[IBIS Ver]   4.1
[File Name]   tms570ls31x_21x_revb_zwt.ibs
[File Rev]   1.0
[Date]   Tue Aug 20 12:42:00 2013
[Source]   Texas Instruments, Inc.
[Notes]   Revision History:
   1.0: initial release, 08/20/2013
   THIS IS RELEASE 1.0,THE CONTENTS ARE SUBJECT TO
   CHANGE WITHOUT PRIOR NOTICE,IF NECESSARY.
[Disclaimer] Please be aware that in the absence of a written agreement
   Texas Instruments(TI) assumes no liability for:
   (1) The accuracy of the IBIS models provided to your company
   (2) The proper functioning of these Models in your design
   or for any resulting applications;or
   (3) Infringement of patents,copyrights or intellectual
   property rights resulting from your use of these models.
   TI provides IBIS Models as a service to our customers and
   therefore reserves the right to limit distribution of the
   Models.
[Copyright]   Property of Texas Instruments Incorporated.
   Unauthorised reproduction and/or distribution is strictly.
   prohibited.
   This product is protected under copyright law and trade
   secret law as an unpublished work.
   Created 2013,(C) Copyright 2013-2014,
   Texas Instruments Incorporated., All Rights Reserved.
   These commodities are under the U.S. Government
   distribution license control.As such,they are not to be
   re-exported without the prior approval of the
   U.S. Department of Commerce.
[Component]   TMS570LS31x/21xZWT
[Manufacturer]   Texas Instruments
[Package]
| variable   typ   min   max
R_pkg   196.67m   3.54953m   570.977m
L_pkg   4.5808nH   0.0479255nH   19.1106nH
C_pkg   1.53489pF   0.703339pF   29.6807pF
[Pin]   signal_name   model_name   R_pin   L_pin   C_pin
|N19	AD1EVT   BQ0210FT	184.966m	4.32413nH	0.998379pF
|V17	AD1IN[01]   IQ0078FT5	151.205m	3.61421nH	1.06433pF
|V18	AD1IN[02]   IQ0078FT5	162.921m	4.0194nH	1.09587pF
|T17	AD1IN[03]   IQ0078FT5	132.107m	2.87623nH	1.02282pF
|U18	AD1IN[04]   IQ0078FT5	150.378m	3.74239nH	0.871765pF
|R17	AD1IN[05]   IQ0078FT5	121.29m   2.64503nH	0.889504pF
|T19	AD1IN[06]   IQ0078FT5	160.561m	4.24427nH	0.832099pF
|V14	AD1IN[07]   IQ0078FT5	124.5m   2.801nH   0.801931pF
|P18	AD1IN[08]_AD2IN[08]	IQ0444FT5	168.416m	3.58257nH	0.854547pF
|W17	AD1IN[09]_AD2IN[09]	IQ0444FT5	176.52m   4.34386nH	0.998673pF
|W14	AD1IN[0]   IQ0078FT5	144.705m	3.56911nH	0.794686pF
|U17	AD1IN[10]_AD2IN[10]	IQ0444FT5	144.94m   3.19721nH	0.980765pF
|U19	AD1IN[11]_AD2IN[11]	IQ0444FT5	171.775m	4.43186nH	0.907619pF
|T16	AD1IN[12]_AD2IN[12]	IQ0444FT5	125.156m	2.59352nH	0.876512pF
|T18	AD1IN[13]_AD2IN[13]	IQ0444FT5	144.177m	3.64898nH	0.839357pF
|R18	AD1IN[14]_AD2IN[14]	IQ0444FT5	165.024m	3.55051nH	0.817191pF
|P19	AD1IN[15]_AD2IN[15]	IQ0444FT5	182.297m	4.13942nH	0.76377pF
|V13	AD1IN[16]_AD2IN[0]	IQ0444FT5	120.853m	2.65468nH	0.725617pF
|U13	AD1IN[17]_AD2IN[01]	IQ0444FT5	100.582m	1.89517nH	0.782711pF
|U14	AD1IN[18]_AD2IN[02]	IQ0444FT5	126.715m	2.5688nH	0.798277pF
|U16	AD1IN[19]_AD2IN[03]	IQ0444FT5	178.504m	4.50312nH	0.988444pF
|U15	AD1IN[20]_AD2IN[04]	IQ0444FT5	119.937m	2.69452nH	0.835124pF
|T15	AD1IN[21]_AD2IN[05]	IQ0444FT5	112.602m	2.37779nH	0.929566pF
|R19	AD1IN[22]_AD2IN[06]	IQ0444FT5	182.419m	4.23756nH	0.798392pF
|R16	AD1IN[23]_AD2IN[07]	IQ0444FT5	142.476m	2.71607nH	0.906429pF
|V15	ADREFHI   BAFTHRU50FT	119.48m		2.9557nH	0.922653pF
|V16	ADREFLO   BAFTHRU50FT	131.598m	3.42945nH	1.00012pF
B10	CAN1RX   BQ0210FT	372.361m	9.36494nH	2.26135pF
A10	CAN1TX			BQ0210FT	363.638m	9.59412nH	2.23947pF
H1	CAN2RX			BQ0210FT	469.673m	12.1979nH	2.87424pF
H2	CAN2TX			BQ0210FT	470.032m	15.4394nH	2.57149pF
M19	CAN3RX			BQ0210FT	401.594m	9.66373nH	2.44197pF
M18	CAN3TX			BQ0210FT	391.963m	9.46214nH	2.55062pF
F17	DMM_CLK			BQ0210FT	153.912m	2.83152nH	1.05028pF
L19	DMM_DATA[0]		BQ0210FT	228.208m	5.86168nH	1.10015pF
L18	DMM_DATA[1]		BQ0210FT	152.021m	3.20684nH	0.961632pF
F16	DMM_NENA		BQ0210FT	109.558m	1.97175nH	1.01071pF
J16	DMM_SYNC		BQ0210FT	131.945m	2.28134nH	1.06088pF
A12	ECLK			BQ0215FT	148.114m	3.69152nH	0.965063pF
D4	EMIF_ADDR[0]		BQ0212FT	205.844m	4.75509nH	1.59007pF
C8	EMIF_ADDR[10]		BQ0212FT	238.21m		5.83758nH	1.71133pF
C9	EMIF_ADDR[11]		BQ0212FT	128.313m	2.08531nH	0.871154pF
C10	EMIF_ADDR[12]		BQ0212FT	123.215m	1.9766nH	0.84691pF
C11	EMIF_ADDR[13]		BQ0212FT	159.315m	3.04056nH	0.957165pF
C12	EMIF_ADDR[14]		BQ0212FT	118.286m	2.54469nH	0.890332pF
C13	EMIF_ADDR[15]		BQ0212FT	126.478m	2.95876nH	0.982603pF
D14	EMIF_ADDR[16]		BQ0212FT	145.307m	2.51953nH	0.973601pF
C14	EMIF_ADDR[17]		BQ0212FT	120.672m	2.47733nH	0.940052pF
D15	EMIF_ADDR[18]		BQ0212FT	111.953m	2.31215nH	0.945399pF
C15	EMIF_ADDR[19]		BQ0212FT	118.554m	2.38397nH	0.981384pF
D5	EMIF_ADDR[1]		BQ0212FT	197.193m	4.27023nH	1.42867pF
C16	EMIF_ADDR[20]		BQ0212FT	150.887m	2.83734nH	1.20313pF
C17	EMIF_ADDR[21]		BQ0212FT	176.774m	3.69908nH	1.27863pF
C4	EMIF_ADDR[6]		BQ0215FT	278.52m   8.56148nH	1.69347pF
C5	EMIF_ADDR[7]		BQ0215FT	304.187m	5.90295nH	2.18684pF
C6	EMIF_ADDR[8]		BQ0215FT	307.858m	6.87831nH	2.13437pF
C7	EMIF_ADDR[9]		BQ0212FT	194.675m	3.98027nH	1.28957pF
D16	EMIF_BA[1]		BQ0215FT	195.47m   4.24161nH	1.29408pF
L3	EMIF_CKE		BQ0212FT	141.86m   2.6218nH	0.864293pF
K3	EMIF_CLK		BQ0212FT	156.267m	3.34722nH	1.22338pF
R4	EMIF_NCAS		BQ0212FT	114.553m	2.02583nH	1.04824pF
N17	EMIF_NCS[0]		BQ0215FT	138.476m	2.73863nH	0.941691pF
L17	EMIF_NCS[2]		BQ0212FT	130.559m	2.55792nH	0.959974pF
K17	EMIF_NCS[3]		BQ0215FT	149.052m	2.77825nH	0.971145pF
M17	EMIF_NCS[4]		BQ0212FT	191.312m	4.44479nH	1.32158pF
R3	EMIF_NRAS		BQ0212FT	148.328m	2.95135nH	1.02744pF
P3	EMIF_NWAIT		BQ0212FT	183.791m	3.30593nH	0.996769pF
D17	EMIF_NWE		BQ0212FT	253.876m	6.55734nH	1.26073pF
R13	ETMDATA[01]		BQ0212FT	124.479m	2.37232nH	0.870061pF
J15	ETMDATA[02]		BQ0212FT	103.911m	1.27754nH	0.953532pF
H15	ETMDATA[03]		BQ0212FT	87.7259m	1.35214nH	1.02626pF
G15	ETMDATA[04]		BQ0212FT	141.552m	2.19702nH	1.13315pF
F15	ETMDATA[05]		BQ0212FT	108.038m	2.13506nH	1.1894pF
E15	ETMDATA[06]		BQ0212FT	150.765m	2.54749nH	1.22031pF
E14	ETMDATA[07]		BQ0212FT	114.504m	1.75736nH	1.21873pF
E9	ETMDATA[08]		BQ0212FT	109.16m   1.64189nH	1.10519pF
E8	ETMDATA[09]		BQ0212FT	144.452m	2.94238nH	1.14497pF
R12	ETMDATA[0]		BQ0212FT	83.6868m	0.985017nH	0.869529pF
E7	ETMDATA[10]		BQ0212FT	214.54m   4.14551nH	1.13678pF
E6	ETMDATA[11]		BQ0212FT	182.856m	3.65155nH	1.40417pF
E13	ETMDATA[12]		BQ0212FT	77.0047m	0.812185nH	0.977195pF
E12	ETMDATA[13]		BQ0212FT	138.149m	1.98855nH	0.973006pF
E11	ETMDATA[14]		BQ0212FT	119.216m	1.28477nH	0.922331pF
E10	ETMDATA[15]		BQ0212FT	118.762m	1.28027nH	0.875094pF
K15	ETMDATA[16]		BQ0212FT	105.18m   1.27303nH	0.910587pF
L15	ETMDATA[17]		BQ0212FT	108.292m	1.30922nH	0.956891pF
M15	ETMDATA[18]		BQ0212FT	146.648m	3.23796nH	1.11212pF
N15	ETMDATA[19]		BQ0212FT	151.481m	2.39079nH	1.04051pF
E5	ETMDATA[20]		BQ0212FT	240.049m	4.95227nH	1.34761pF
F5	ETMDATA[21]		BQ0212FT	200.894m	3.43241nH	1.2936pF
G5	ETMDATA[22]		BQ0212FT	113.089m	1.56898nH	1.27784pF
K5	ETMDATA[23]		BQ0212FT	159.632m	2.73815nH	1.23965pF
L5	ETMDATA[24]		BQ0212FT	107.976m	1.33411nH	0.987891pF
M5	ETMDATA[25]		BQ0212FT	158.798m	1.84169nH	0.949294pF
N5	ETMDATA[26]		BQ0212FT	104.885m	1.27901nH	0.956427pF
P5	ETMDATA[27]		BQ0212FT	111.148m	1.31516nH	0.975979pF
R5	ETMDATA[28]		BQ0212FT	99.3475m	1.3689nH	1.06642pF
R6	ETMDATA[29]		BQ0212FT	97.4645m	1.43736nH	1.09879pF
R7	ETMDATA[30]		BQ0212FT	124.403m	1.9796nH	0.99492pF
R8	ETMDATA[31]		BQ0212FT	104.139m	1.40991nH	0.846212pF
R9	ETMTRACECLKIN		BQ0212FT	121.779m	1.22371nH	0.853714pF
R10	ETMTRACECLKOUT		BQ0212FT	142.063m	1.98785nH	0.918845pF
R11	ETMTRACECTL		BQ0212FT	190.384m	2.91831nH	0.965226pF
|J5	FLTP1			BAFTHRU15VFT   149.492m	2.20118nH	1.45838pF
|H5	FLTP2			BAFTHRU8VFT   165.991m	2.9168nH	1.52069pF
A15	FRAYRX1			IQ0442FT_40P60P	239.448m	7.10463nH	1.25424pF
A8	FRAYRX2			IQ0442FT_40P60P	258.134m	7.31683nH	1.55084pF
B15	FRAYTX1			OQ0112FT	304.358m	8.80599nH	1.6535pF
B8	FRAYTX2			OQ0112FT	226.744m	5.13131nH	1.43502pF
B16	FRAYTXEN1		OQ0112FT	349.226m	11.4289nH	1.99559pF
B9	FRAYTXEN2		OQ0112FT	258.966m	6.63073nH	1.55419pF
A5	GIOA[0]			BQ0210FT	190.079m	4.2665nH	1.13619pF
C2	GIOA[1]			BQ0210FT	185.052m	4.37032nH	1.10133pF
C1	GIOA[2]			BQ0215FT	218.526m	6.21769nH	1.17667pF
E1	GIOA[3]			BQ0210FT	210.54m   5.74448nH	1.10806pF
A6	GIOA[4]			BQ0210FT	385.739m	11.963nH	2.08522pF
B5	GIOA[5]			BQ0210FT	280.374m	5.73605nH	2.17708pF
H3	GIOA[6]			BQ0210FT	161.443m	4.06305nH	1.16964pF
M1	GIOA[7]			BQ0210FT	216.429m	4.60646nH	0.861283pF
M2	GIOB[0]			BQ0215FT	344.684m	8.17302nH	2.2998pF
K2	GIOB[1]			BQ0215FT	513.961m	16.8626nH	2.48021pF
F2	GIOB[2]			BQ0210FT	256.042m	6.4832nH	1.48887pF
W10	GIOB[3]			BQ0210FT	564.754m	12.7444nH	3.11943pF
G1	GIOB[4]			BQ0210FT	207.863m	4.2053nH	1.17746pF
G2	GIOB[5]			BQ0210FT	176.17m   4.21454nH	1.07738pF
J2	GIOB[6]			BQ0210FT	249.666m	4.98691nH	1.1261pF
F1	GIOB[7]			BQ0210FT	431.321m	11.1455nH	2.1899pF
|L2	KELVIN_GND		GND   144.49m   3.36085nH	0.855052pF
A7	LINRX			BQ0210FT	164.093m	3.51713nH	0.789652pF
B7	LINTX			BQ0210FT	149.514m	3.76138nH	0.974205pF
F18	MIBSPI1CLK		BQ0211FT	209.432m	5.11407nH	1.36171pF
R2	MIBSPI1NCS[0]		BQ0215FT	438.232m	9.65193nH	2.73624pF
F3	MIBSPI1NCS[1]		BQ0215FT	249.337m	5.36744nH	1.38728pF
G3	MIBSPI1NCS[2]		BQ0215FT	570.977m	19.1106nH	3.13273pF
J3	MIBSPI1NCS[3]		BQ0210FT	533.925m	18.0739nH	2.91425pF
G19	MIBSPI1NENA		BQ0210FT	222.255m	5.67898nH	1.17997pF
F19	MIBSPI1SIMO		BQ0211FT	255.952m	7.3408nH	1.63182pF
G18	MIBSPI1SOMI		BQ0211FT	248.638m	6.78288nH	1.35142pF
V9	MIBSPI3CLK		BQ0211FT	143.966m	2.67746nH	0.710513pF
V10	MIBSPI3NCS[0]		BQ0210FT	159.677m	2.96343nH	0.703339pF
V5	MIBSPI3NCS[1]		BQ0215FT	129.845m	2.82102nH	0.865993pF
B2	MIBSPI3NCS[2]		BQ0210FT	197.146m	4.5376nH	1.01987pF
C3	MIBSPI3NCS[3]		BQ0210FT	173.194m	3.67063nH	1.03815pF
W9	MIBSPI3NENA		BQ0210FT	174.924m	3.75475nH	0.75194pF
W8	MIBSPI3SIMO		BQ0211FT	174.737m	3.8999nH	0.788207pF
V8	MIBSPI3SOMI		BQ0211FT	157.163m	3.04464nH	0.770715pF
H19	MIBSPI5CLK		BQ0212FT	172.551m	4.02962nH	1.0456pF
E19	MIBSPI5NCS[0]		BQ0210FT	434.627m	9.75226nH	2.8982pF
B6	MIBSPI5NCS[1]		BQ0210FT	125.385m	2.81804nH	0.998305pF
W6	MIBSPI5NCS[2]		BQ0210FT	137.701m	3.4368nH	0.777293pF
T12	MIBSPI5NCS[3]		BQ0210FT	88.9463m	1.39nH   0.752235pF
H18	MIBSPI5NENA		BQ0210FT	172.956m	3.92446nH	1.06336pF
J19	MIBSPI5SIMO[0]		BQ0212FT	230.569m	5.55483nH	1.25878pF
E16	MIBSPI5SIMO[1]		BQ0212FT	113.502m	2.01142nH	1.12975pF
H17	MIBSPI5SIMO[2]		BQ0212FT	147.332m	2.72568nH	1.04308pF
G17	MIBSPI5SIMO[3]		BQ0212FT	136.981m	2.49108nH	1.02895pF
J18	MIBSPI5SOMI[0]		BQ0212FT	150.574m	3.17152nH	1.01665pF
E17	MIBSPI5SOMI[1]		BQ0212FT	228.929m	5.42812nH	1.37918pF
H16	MIBSPI5SOMI[2]		BQ0212FT	140.961m	3.01931nH	1.21316pF
G16	MIBSPI5SOMI[3]		BQ0212FT	112.489m	1.67887nH	1.04781pF
B14	NERROR			BQ0212FT	138.758m	3.33213nH	1.04178pF
V2	NHET1[01]		BQ0215FT	338.409m	9.38218nH	1.48365pF
W5	NHET1[02]		BQ0215FT	248.268m	6.84186nH	1.56548pF
U1	NHET1[03]		BQ0215FT	293.29m   7.89763nH	1.33136pF
B12	NHET1[04]		BQ0210FT	384.915m	8.28491nH	2.24703pF
V6	NHET1[05]		BQ0215FT	222.182m	5.35492nH	1.44554pF
W3	NHET1[06]		BQ0210FT	169.477m	4.54954nH	0.866005pF
T1	NHET1[07]		BQ0215FT	177.683m	4.12802nH	0.940453pF
E18	NHET1[08]		BQ0215FT	169.207m	3.50595nH	1.02982pF
V7	NHET1[09]		BQ0215FT	164.378m	3.85974nH	1.41149pF
K18	NHET1[0]		BQ0215FT	502.921m	10.4825nH	2.67359pF
D19	NHET1[10]		BQ0215FT	284.952m	7.64309nH	1.46318pF
E3	NHET1[11]		BQ0210FT	142.81m   2.72692nH	1.13821pF
B4	NHET1[12]		BQ0210FT	363.144m	10.8745nH	1.72677pF
N2	NHET1[13]		BQ0210FT	272.616m	7.56634nH	1.52295pF
A11	NHET1[14]		BQ0215FT	171.543m	3.6018nH	0.779645pF
N1	NHET1[15]		BQ0210FT	279.581m	8.1671nH	1.60856pF
A4	NHET1[16]		BQ0210FT	175.761m	4.52014nH	1.03411pF
A13	NHET1[17]		BQ0210FT	241.835m	6.51525nH	1.41446pF
J1	NHET1[18]		BQ0210FT	265.215m	6.2119nH	2.32332pF
B13	NHET1[19]		BQ0210FT	156.895m	3.0638nH	0.861316pF
P2	NHET1[20]		BQ0210FT	312.077m	7.55077nH	2.22707pF
H4	NHET1[21]		BQ0210FT	111.925m	1.75875nH	1.25067pF
B3	NHET1[22]		BQ0215FT	350.67m   11.5381nH	1.82498pF
J4	NHET1[23]		BQ0210FT	123.48m   1.96598nH	1.02514pF
P1	NHET1[24]		BQ0210FT	396.061m	10.0857nH	2.38747pF
M3	NHET1[25]		BQ0210FT	170.639m	3.82685nH	1.09905pF
A14	NHET1[26]		BQ0210FT	449.316m	15.0385nH	2.06763pF
A9	NHET1[27]		BQ0210FT	168.919m	3.59624nH	0.808161pF
K19	NHET1[28]		BQ0215FT	259.145m	7.72222nH	1.78386pF
A3	NHET1[29]		BQ0210FT	308.914m	7.89948nH	1.44571pF
B11	NHET1[30]		BQ0215FT	150.979m	3.75274nH	0.934869pF
J17	NHET1[31]		BQ0210FT	124.28m   2.62385nH	0.959855pF
W7	NPORRST			IQ0087FT	133.059m	3.12687nH	0.709599pF
B17	NRST			BQ0414FT	182.53m   4.97021nH	1.03603pF
D18	NTRST			IQ0087FT	152.716m	2.92701nH	1.15626pF
|K1	OSCIN			IOSCHF33FTHY_NI	182.979m	4.30943nH	0.900278pF
|L1	OSCOUT			OOSCHF33FT	177.748m	4.18486nH	0.900586pF
A16	RTCK			OQ0112FT	162.129m	4.03402nH	0.892402pF
E2	SPI2CLK			BQ0215FT	375.515m	9.50242nH	2.50953pF
N3	SPI2NCS[0]		BQ0210FT	173.134m	3.45939nH	1.0953pF
D3	SPI2NENA		BQ0210FT	343.918m	8.21745nH	2.25067pF
D1	SPI2SIMO		BQ0215FT	385.568m	10.3648nH	2.42637pF
D2	SPI2SOMI		BQ0215FT	383.751m	9.92658nH	2.49432pF
B18	TCK			IQ0079FT	176.229m	4.16813nH	1.08376pF
A17	TDI			BQ0192FT	194.968m	4.09791nH	1.12659pF
C18	TDO			BQ0192FT	165.391m	3.63759nH	1.18983pF
U2	TEST			BQ0213FT	192.031m	4.40728nH	1.0986pF
C19	TMS			BQ0192FT	176.949m	3.26783nH	1.07488pF
|VCC	VCC			POWER		4.66918m	0.0841554nH	13.8474pF
|VCCAD	VCCAD			POWER		190.835m	4.78259nH	1.13553pF
|VCCIO	VCCIO			POWER		3.75816m	0.0479255nH	15.3635pF
|F8	VCCP			POWER		63.0872m	0.884806nH	1.16442pF
|P11	VCCPLL			POWER		62.0258m	0.876174nH	1.035pF
|VSS	VSS			GND		3.54953m	0.0778735nH	29.6807pF
|VSSAD	VSSAD			GND		112.521m	3.46255nH	3.01863pF
[Model Selector] BQ0192FT
BQ0192FT_PZ_3P3  Cell operated at 3.3(nom)
|BQ0192FT_PZ_3P3; PUPD_OFF
BQ0192FT_PU_3P3  Cell operated at 3.3(nom)
|BQ0192FT_PU_3P3; PULLUP_ON
BQ0192FT_PD_3P3  Cell operated at 3.3(nom)
|BQ0192FT_PD_3P3; PULLDOWN_ON
[Model Selector] BQ0210FT
BQ0210FT_PZ_3P3  Cell operated at 3.3(nom)
|BQ0210FT_PZ_3P3; PUPD_OFF
BQ0210FT_PU_3P3  Cell operated at 3.3(nom)
|BQ0210FT_PU_3P3; PULLUP_ON
BQ0210FT_PD_3P3  Cell operated at 3.3(nom)
|BQ0210FT_PD_3P3; PULLDOWN_ON
[Model Selector] BQ0211FT
BQ0211FT_PZ_3P3  Cell operated at 3.3(nom)
|BQ0211FT_PZ_3P3; PUPD_OFF
BQ0211FT_PU_3P3  Cell operated at 3.3(nom)
|BQ0211FT_PU_3P3; PULLUP_ON
BQ0211FT_PD_3P3  Cell operated at 3.3(nom)
|BQ0211FT_PD_3P3; PULLDOWN_ON
[Model Selector] BQ0212FT
BQ0212FT_PZ_3P3  Cell operated at 3.3(nom)
|BQ0212FT_PZ_3P3; PUPD_OFF
BQ0212FT_PU_3P3  Cell operated at 3.3(nom)
|BQ0212FT_PU_3P3; PULLUP_ON
BQ0212FT_PD_3P3  Cell operated at 3.3(nom)
|BQ0212FT_PD_3P3; PULLDOWN_ON
[Model Selector] BQ0213FT
BQ0213FT_PZ_3P3  Cell operated at 3.3(nom)
|BQ0213FT_PZ_3P3; PULLDOWN_OFF
BQ0213FT_PD_3P3  Cell operated at 3.3(nom)
|BQ0213FT_PD_3P3; PULLDOWN_ON
[Model Selector] BQ0215FT
BQ0215FT_PZ_3P3  Cell operated at 3.3(nom)
|BQ0215FT_PZ_3P3; PUPD_OFF
BQ0215FT_PU_3P3  Cell operated at 3.3(nom)
|BQ0215FT_PU_3P3; PULLUP_ON
BQ0215FT_PD_3P3  Cell operated at 3.3(nom)
|BQ0215FT_PD_3P3; PULLDOWN_ON
[Model Selector] BQ0414FT
BQ0414FT_PZ_3P3  Cell operated at 3.3(nom)
|BQ0414FT_PZ_3P3; PUPD_OFF
BQ0414FT_PU_3P3  Cell operated at 3.3(nom)
|BQ0414FT_PU_3P3; PULLUP_ON
BQ0414FT_PD_3P3  Cell operated at 3.3(nom)
|BQ0414FT_PD_3P3; PULLDOWN_ON
[Model Selector] IQ0079FT
IQ0079FT_PZ_3P3  Cell operated at 3.3(nom)
|IQ0079FT_PZ_3P3; PUPD_OFF
IQ0079FT_PU_3P3  Cell operated at 3.3(nom)
|IQ0079FT_PU_3P3; PULLUP_ON
IQ0079FT_PD_3P3  Cell operated at 3.3(nom)
|IQ0079FT_PD_3P3; PULLDOWN_ON
[Model Selector] IQ0087FT
IQ0087FT_PZ_3P3  Cell operated at 3.3(nom)
|IQ0087FT_PZ_3P3; PULLDOWN_OFF
IQ0087FT_PD_3P3  Cell operated at 3.3(nom)
|IQ0087FT_PD_3P3; PULLDOWN_ON
[Model Selector] IQ0442FT_40P60P
0442FT_40P60P_PZ_3P3  Cell operated at 3.3(nom)
|IQ0442FT_40P60P_PZ_3P3; PUPD_OFF
2FT_40P60P_PU_3P3  Cell operated at 3.3(nom)
|IQ0442FT_40P60P_PU_3P3; PULLUP_ON
2FT_40P60P_PD_3P3  Cell operated at 3.3(nom)
| Models and submodels in the file (29): BQ0192FT_PZ_3P3 (I/O), BQ0192FT_PU_3P3 (I/O), BQ0192FT_PD_3P3 (I/O), BQ0210FT_PZ_3P3 (I/O), BQ0210FT_PU_3P3 (I/O), BQ0210FT_PD_3P3 (I/O), BQ0211FT_PZ_3P3 (I/O), BQ0211FT_PU_3P3 (I/O), BQ0211FT_PD_3P3 (I/O), BQ0212FT_PZ_3P3 (I/O), BQ0212FT_PU_3P3 (I/O), BQ0212FT_PD_3P3 (I/O), BQ0213FT_PZ_3P3 (I/O), BQ0213FT_PD_3P3 (I/O), BQ0215FT_PZ_3P3 (I/O), BQ0215FT_PU_3P3 (I/O), BQ0215FT_PD_3P3 (I/O), BQ0414FT_PZ_3P3 (I/O), BQ0414FT_PU_3P3 (I/O), BQ0414FT_PD_3P3 (I/O), IQ0079FT_PZ_3P3 (Input), IQ0079FT_PU_3P3 (Input), IQ0079FT_PD_3P3 (Input), IQ0087FT_PZ_3P3 (Input), IQ0087FT_PD_3P3 (Input), 0442FT_40P60P_PZ_3P3 (Input), 2FT_40P60P_PU_3P3 (Input), 2FT_40P60P_PD_3P3 (Input), OQ0112FT (3-state)
